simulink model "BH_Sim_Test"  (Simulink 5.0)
settings: Solver=ode4  StartTime=0.0  StopTime=inf  FixedStep=0.001  RelTol=1e-3
undefined symbols (not defined in the file or in its folder): com, uint
libraries: xpclib x8

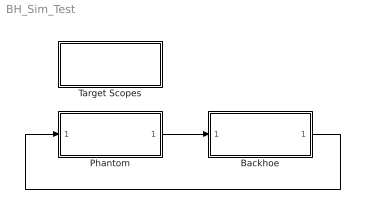
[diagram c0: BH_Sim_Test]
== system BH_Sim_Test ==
  Backhoe : Subsystem
  Phantom : Subsystem
  Target Scopes : Subsystem
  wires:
  Backhoe/1(yb) -> Phantom/1(Yb)
  Phantom/1(Yb_Desired) -> Backhoe/1(yp)

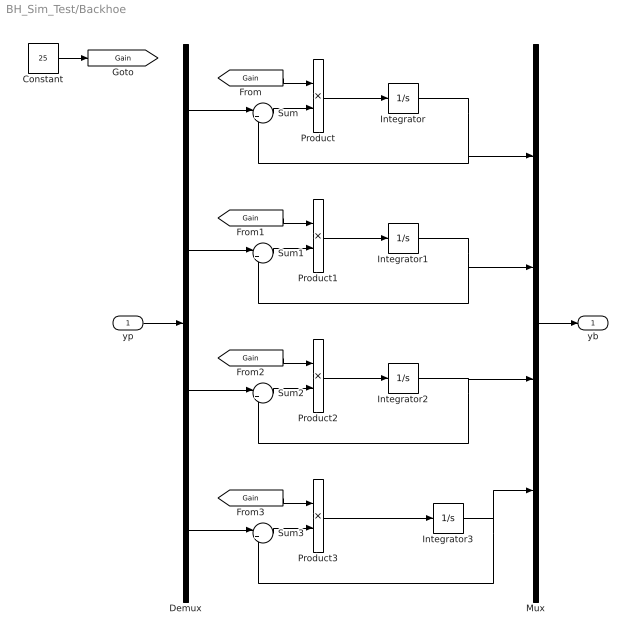
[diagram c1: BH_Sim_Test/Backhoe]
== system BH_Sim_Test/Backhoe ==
  yp : Inport
  Constant : Constant  Value=25
  Demux : Demux
  Integrator{,1..3} (4 alike) : Integrator
  Mux : Mux
  Product{,1..3} (4 alike) : Product
  Sum{,1..3} (4 alike) : Sum  Inputs=|+-
  yb : Outport
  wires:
  Constant/1 -> [Gain]
  yp/1 -> Demux/1
  Demux/1 -> Sum/1
  Sum/1 -> Product/2
  [Gain] -> Product/1
  Product/1 -> Integrator/1
  Integrator/1 -> Mux/1, Sum/2
  Demux/2 -> Sum1/1
  Sum1/1 -> Product1/2
  [Gain] -> Product1/1
  Product1/1 -> Integrator1/1
  Integrator1/1 -> Sum1/2, Mux/2
  Sum2/1 -> Product2/2
  [Gain] -> Product2/1
  Product2/1 -> Integrator2/1
  Integrator2/1 -> Sum2/2, Mux/3
  Demux/3 -> Sum2/1
  Sum3/1 -> Product3/2
  [Gain] -> Product3/1
  Demux/4 -> Sum3/1
  Integrator3/1 -> Sum3/2, Mux/4
  Product3/1 -> Integrator3/1
  Mux/1 -> yb/1

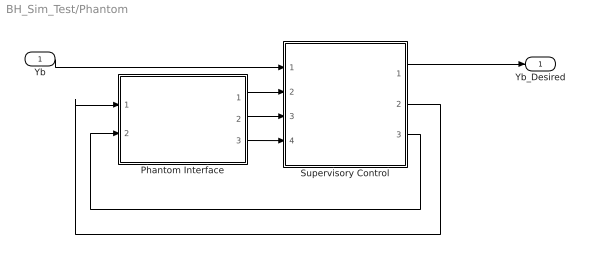
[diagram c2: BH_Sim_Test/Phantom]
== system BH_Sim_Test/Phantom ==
  Yb : Inport
  Phantom Interface : Subsystem
  Supervisory Control : Subsystem
  Yb_Desired : Outport
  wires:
  Yb/1 -> Supervisory Control/1(Y_Bh)
  Supervisory Control/1(Y_Bh_ref) -> Yb_Desired/1
  Phantom Interface/1("Yp ") -> Supervisory Control/2(Y_Ph_In)
  Phantom Interface/2(Ph_Time) -> Supervisory Control/3(Ph_Time)
  Phantom Interface/3(Ph_Flag) -> Supervisory Control/4(Ph Flag)
  Supervisory Control/3(OUt_Flag) -> Phantom Interface/2(Bh_Flag)
  Supervisory Control/2(Send2Ph) -> Phantom Interface/1(Yb)

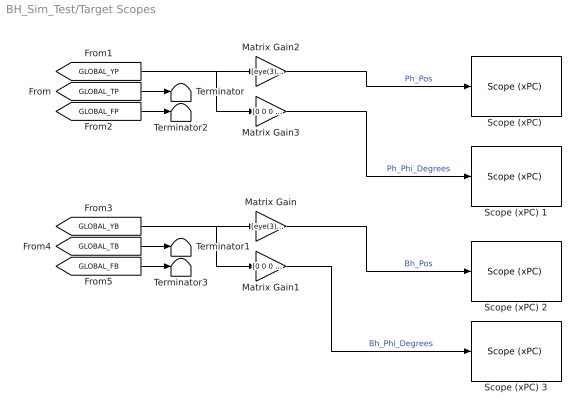
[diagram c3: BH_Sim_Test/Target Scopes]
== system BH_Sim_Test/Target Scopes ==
  Matrix Gain : Gain  Gain=[eye(3) zeros(3,1)]  Multiplication=Matrix(K*u)
  Matrix Gain1 : Gain  Gain=[0 0 0 180/pi]  Multiplication=Matrix(K*u)
  Matrix Gain2 : Gain  Gain=[eye(3) zeros(3,1)]  Multiplication=Matrix(K*u)
  Matrix Gain3 : Gain  Gain=[0 0 0 180/pi]  Multiplication=Matrix(K*u)
  "Scope (xPC) " : xpclib/Misc./Scope (xPC)   scopeno=1  scopetype=Target  viewmode=Graphical redraw  grid=on  ylimits=[0,0]  autostart=on  nosamples=1000  noprepostsamples=0  interleave=1  triggermode=FreeRun  triggersignal=1  triggerlevel=0.0  triggerslope=either  triggerscope=1  triggersample=0
  Scope (xPC) 1 : xpclib/Misc./Scope (xPC)   scopeno=2  scopetype=Target  viewmode=Graphical redraw  grid=on  ylimits=[-120,90]  autostart=on  nosamples=1000  noprepostsamples=0  interleave=1  triggermode=FreeRun  triggersignal=1  triggerlevel=0.0  triggerslope=either  triggerscope=1  triggersample=0
  Scope (xPC) 2 : xpclib/Misc./Scope (xPC)   scopeno=3  scopetype=Target  viewmode=Graphical redraw  grid=on  ylimits=[0,0]  autostart=on  nosamples=1000  noprepostsamples=0  interleave=1  triggermode=FreeRun  triggersignal=1  triggerlevel=0.0  triggerslope=either  triggerscope=1  triggersample=0
  Scope (xPC) 3 : xpclib/Misc./Scope (xPC)   scopeno=4  scopetype=Target  viewmode=Graphical redraw  grid=on  ylimits=[-120,90]  autostart=on  nosamples=1000  noprepostsamples=0  interleave=1  triggermode=FreeRun  triggersignal=1  triggerlevel=0.0  triggerslope=either  triggerscope=1  triggersample=0
  Terminator{,1..3} (4 alike) : Terminator
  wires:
  [GLOBAL_TP] -> Terminator/1
  [GLOBAL_TB] -> Terminator1/1
  [GLOBAL_FP] -> Terminator2/1
  [GLOBAL_FB] -> Terminator3/1
  [GLOBAL_YB] -> Matrix Gain/1, Matrix Gain1/1
  [GLOBAL_YP] -> Matrix Gain2/1, Matrix Gain3/1
  Matrix Gain2/1 -> "Scope (xPC) "/1  "Ph_Pos"
  Matrix Gain3/1 -> Scope (xPC) 1/1  "Ph_Phi_Degrees"
  Matrix Gain/1 -> Scope (xPC) 2/1  "Bh_Pos"
  Matrix Gain1/1 -> Scope (xPC) 3/1  "Bh_Phi_Degrees"

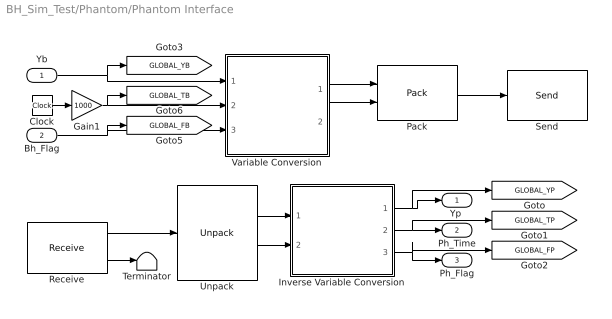
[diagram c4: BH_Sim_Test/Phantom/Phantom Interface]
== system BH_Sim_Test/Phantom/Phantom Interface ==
  Yb : Inport
  Bh_Flag : Inport  Port=2
  Clock : Clock
  Gain1 : Gain  Gain=1000  ShowAdditionalParam=on  OutDataTypeMode=Specify via dialog  OutDataType=uint(32)
  Inverse Variable Conversion : Subsystem
  Pack : xpclib/UDP/Pack  datatypes={'double','uint32'}  byteAlign=8
  Receive : xpclib/UDP/Receive  ipAddress=0.0.0.0  ipPort=com.Ph2Bh_Port  width=com.Ph2Bh_Bytes  sampletime=Sampling_Time
  Send : xpclib/UDP/Send  ipAddress=com.SendIP  ipPort=com.Bh2Ph_Port  sampletime=Sampling_Time
  Terminator : Terminator
  Unpack : xpclib/UDP/Unpack  dimensions=com.Ph2Bh_Port_Dim  datatypes={'double','uint32'}  byteAlign=8
  Variable Conversion : Subsystem
  "Yp " : Outport
  Ph_Time : Outport  Port=2
  Ph_Flag : Outport  Port=3
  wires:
  Receive/2 -> Terminator/1
  Receive/1 -> Unpack/1
  Pack/1 -> Send/1
  Yb/1 -> Variable Conversion/1(Yb), [GLOBAL_YB]
  Bh_Flag/1 -> [GLOBAL_FB], Variable Conversion/3(Bh_Flag)
  Inverse Variable Conversion/1(Yp) -> "Yp "/1, [GLOBAL_YP]
  Unpack/1 -> Inverse Variable Conversion/1(doubles)
  Inverse Variable Conversion/3(Ph_Flag) -> Ph_Flag/1, [GLOBAL_FP]
  Inverse Variable Conversion/2(Ph_Time) -> Ph_Time/1, [GLOBAL_TP]
  Unpack/2 -> Inverse Variable Conversion/2(uint32s)
  Variable Conversion/2(uint32s) -> Pack/2
  Variable Conversion/1(doubles) -> Pack/1
  Clock/1 -> Gain1/1
  Gain1/1 -> [GLOBAL_TB], Variable Conversion/2(Bh_Time)

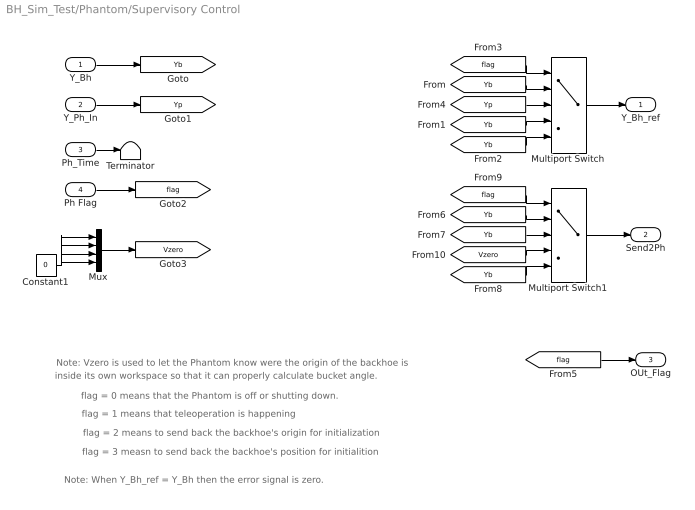
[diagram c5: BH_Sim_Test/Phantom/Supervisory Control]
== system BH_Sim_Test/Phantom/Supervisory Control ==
  note: Note: Vzero is used to let the Phantom know were the origin of the backhoe is
  note: flag = 0 means that the Phantom is off or shutting down.
  note: flag = 3 measn to send back the backhoe's position for initialition
  note: inside its own workspace so that it can properly calculate bucket angle.
  note: flag = 1 means that teleoperation is happening
  note: flag = 2 means to send back the backhoe's origin for initialization
  note: Note: When Y_Bh_ref = Y_Bh then the error signal is zero.
  Y_Bh : Inport
  Y_Ph_In : Inport  Port=2
  Ph_Time : Inport  Port=3
  Ph Flag : Inport  Port=4
  Constant1 : Constant  Value=0
  Multiport Switch : MultiPortSwitch  ShowAdditionalParam=on  zeroidx=on
  Multiport Switch1 : MultiPortSwitch  ShowAdditionalParam=on  zeroidx=on
  Mux : Mux
  Terminator : Terminator
  Y_Bh_ref : Outport
  Send2Ph : Outport  Port=2
  OUt_Flag : Outport  Port=3
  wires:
  Ph_Time/1 -> Terminator/1
  [flag] -> OUt_Flag/1
  Y_Ph_In/1 -> [Yp]
  Y_Bh/1 -> [Yb]
  Ph Flag/1 -> [flag]
  Constant1/1 -> Mux/1, Mux/4, Mux/3, Mux/2
  Mux/1 -> [Vzero]
  [Yb] -> Multiport Switch/2
  [Yb] -> Multiport Switch/4
  [Yb] -> Multiport Switch/5
  Multiport Switch/1 -> Y_Bh_ref/1
  [flag] -> Multiport Switch/1
  [Yp] -> Multiport Switch/3
  [Yb] -> Multiport Switch1/2
  [Vzero] -> Multiport Switch1/4
  [Yb] -> Multiport Switch1/5
  [flag] -> Multiport Switch1/1
  [Yb] -> Multiport Switch1/3
  Multiport Switch1/1 -> Send2Ph/1

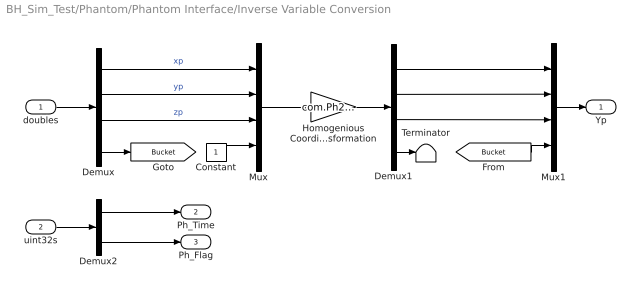
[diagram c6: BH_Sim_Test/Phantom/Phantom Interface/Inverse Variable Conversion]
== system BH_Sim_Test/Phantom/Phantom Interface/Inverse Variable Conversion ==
  doubles : Inport
  uint32s : Inport  Port=2
  Constant : Constant
  Demux : Demux
  Demux1 : Demux
  Demux2 : Demux  Outputs=2
  Homogenious Coordinate Transformation : Gain  Gain=com.Ph2Bh_Transform  Multiplication=Matrix(K*u)  ShowAdditionalParam=on
  Mux : Mux
  Mux1 : Mux
  Terminator : Terminator
  Yp : Outport
  Ph_Time : Outport  Port=2
  Ph_Flag : Outport  Port=3
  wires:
  doubles/1 -> Demux/1
  Demux/1 -> Mux/1  "xp"
  Demux/2 -> Mux/2  "yp"
  Demux/3 -> Mux/3  "zp"
  Mux/1 -> Homogenious Coordinate Transformation/1
  Demux2/1 -> Ph_Time/1
  Demux2/2 -> Ph_Flag/1
  Demux/4 -> [Bucket]
  Constant/1 -> Mux/4
  Homogenious Coordinate Transformation/1 -> Demux1/1
  Demux1/4 -> Terminator/1
  Mux1/1 -> Yp/1
  Demux1/3 -> Mux1/3
  Demux1/2 -> Mux1/2
  Demux1/1 -> Mux1/1
  [Bucket] -> Mux1/4
  uint32s/1 -> Demux2/1

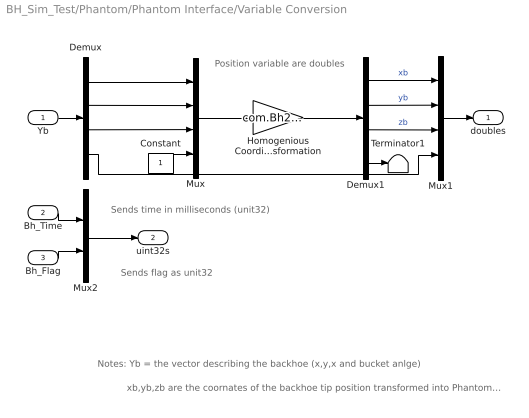
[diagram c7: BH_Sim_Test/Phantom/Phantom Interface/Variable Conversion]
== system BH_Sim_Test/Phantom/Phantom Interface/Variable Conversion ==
  note: Sends time in milliseconds (unit32)
  note: Sends flag as unit32
  note: Position variable are doubles
  note: Notes: Yb = the vector describing the backhoe (x,y,x and bucket anlge)
  note: xb,yb,zb are the coornates of the backhoe tip position transformed into Phantom coordinates
  Yb : Inport
  Bh_Time : Inport  Port=2
  Bh_Flag : Inport  Port=3
  Constant : Constant
  Demux : Demux
  Demux1 : Demux
  Homogenious Coordinate Transformation : Gain  Gain=com.Bh2Ph_Transform  Multiplication=Matrix(K*u)  ShowAdditionalParam=on
  Mux : Mux
  Mux1 : Mux
  Mux2 : Mux  Inputs=2
  Terminator1 : Terminator
  doubles : Outport
  uint32s : Outport  Port=2
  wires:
  Demux/1 -> Mux/1
  Demux/2 -> Mux/2
  Yb/1 -> Demux/1
  Demux/3 -> Mux/3
  Bh_Flag/1 -> Mux2/2
  Constant/1 -> Mux/4
  Homogenious Coordinate Transformation/1 -> Demux1/1
  Mux/1 -> Homogenious Coordinate Transformation/1
  Demux1/1 -> Mux1/1  "xb"
  Demux1/2 -> Mux1/2  "yb"
  Demux1/3 -> Mux1/3  "zb"
  Demux1/4 -> Terminator1/1
  Bh_Time/1 -> Mux2/1
  Mux2/1 -> uint32s/1
  Mux1/1 -> doubles/1
  Demux/4 -> Mux1/4
